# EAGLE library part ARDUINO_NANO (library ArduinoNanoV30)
Arduino Nano V3.0 Module Overview: The Arduino Nano is a small, complete, and breadboard-friendly board based on the ATmega328 (Arduino Nano 3.x) or ATmega168 (Arduino Nano 2.x). It has more or less the same functionality of the Arduino Duemilanove, but in a different package. It lacks only a DC power jack, and works with a Mini-B USB cable instead of a standard one. The Nano was designed and is being produced by Gravitech. General specifications: Item Value Microcontroller Atmel ATmega168 or ATmega328 Operating Voltage (logic level) 5 V Input Voltage (recommended) 7-12 V Input Voltage (limits) 6-20 V Digital I/O Pins 14 (of which 6 provide PWM output) Analog Input Pins 8 DC Current per I/O Pin 40 mA Flash Memory 16 KB (ATmega168) or 32 KB (ATmega328) of which 2 KB used by bootloader SRAM 1 KB (ATmega168) or 2 KB (ATmega328) EEPROM 512 bytes (ATmega168) or 1 KB (ATmega328) Clock Speed 16 MHz Dimensions (Inches) 0.73" x 1.70" Dimensions (mm) 18mm x 45mm Overall height About 9 mm (not including pins) Weigth 5 g Power: The Arduino Nano can be powered via the Mini-B USB connection, 6-20V unregulated external power supply (pin 30), or 5V regulated external power supply (pin 27). The power source is automatically selected to the highest voltage source. Memory: The ATmega168 has 16 KB of flash memory for storing code (of which 2 KB is used for the bootloader); the ATmega328 has 32 KB, (also with 2 KB used for the bootloader). The ATmega168 has 1 KB of SRAM and 512 bytes of EEPROM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
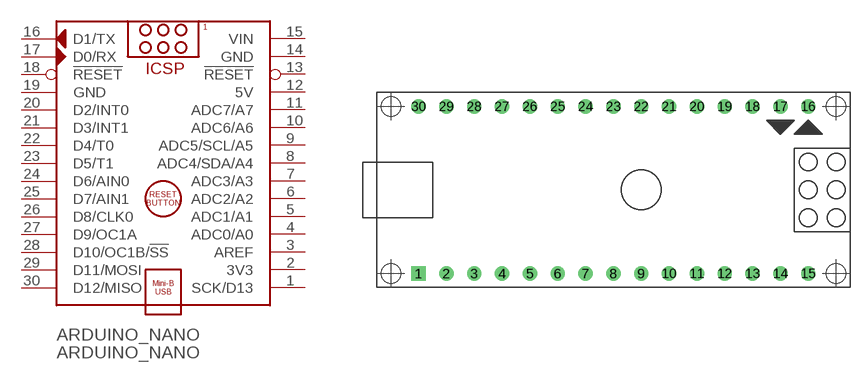
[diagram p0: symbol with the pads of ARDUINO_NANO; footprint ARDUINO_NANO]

Designator prefix ARDUINO_NANO

## ARDUINO_NANO  [ARDUINO_NANO]
1  SCK/D13
2  3V3  out
3  AREF  in
4  ADC0/A0
5  ADC1/A1
6  ADC2/A2
7  ADC3/A3
8  ADC4/SDA/A4
9  ADC5/SCL/A5
10  ADC6/A6
11  ADC7/A7
12  5V  pwr
13  !RESET  in
14  GND  pwr
15  VIN  pwr
16  D1/TX
17  D0/RX
18  !RESET  in
19  GND  pwr
20  D2/INT0
21  D3/INT1
22  D4/T0
23  D5/T1
24  D6/AIN0
25  D7/AIN1
26  D8/CLK0
27  D9/OC1A
28  D10/OC1B/!SS
29  D11/MOSI
30  D12/MISO

## Footprint ARDUINO_NANO (pad centres in mm)
Arduino Nano V3.0 Module The Nano was designed and is being produced by Gravitech.
drill 0.8 square: 1 -20.32,-7.62
drill 0.8: 2 -17.78,-7.62; 3 -15.24,-7.62; 4 -12.7,-7.62; 5 -10.16,-7.62; 6 -7.62,-7.62; 7 -5.08,-7.62; 8 -2.54,-7.62; 9 0,-7.62; 10 2.54,-7.62; 11 5.08,-7.62; 12 7.62,-7.62; 13 10.16,-7.62; 14 12.7,-7.62; 15 15.24,-7.62; 16 15.24,7.62; 17 12.7,7.62; 18 10.16,7.62; 19 7.62,7.62; 20 5.08,7.62; 21 2.54,7.62; 22 0,7.62; 23 -2.54,7.62; 24 -5.08,7.62; 25 -7.62,7.62; 26 -10.16,7.62; 27 -12.7,7.62; 28 -15.24,7.62; 29 -17.78,7.62; 30 -20.32,7.62
hole 1.778 at -22.86,-7.62
hole 1.778 at -22.86,7.62
hole 1.778 at 17.78,7.62
hole 1.778 at 17.78,-7.62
